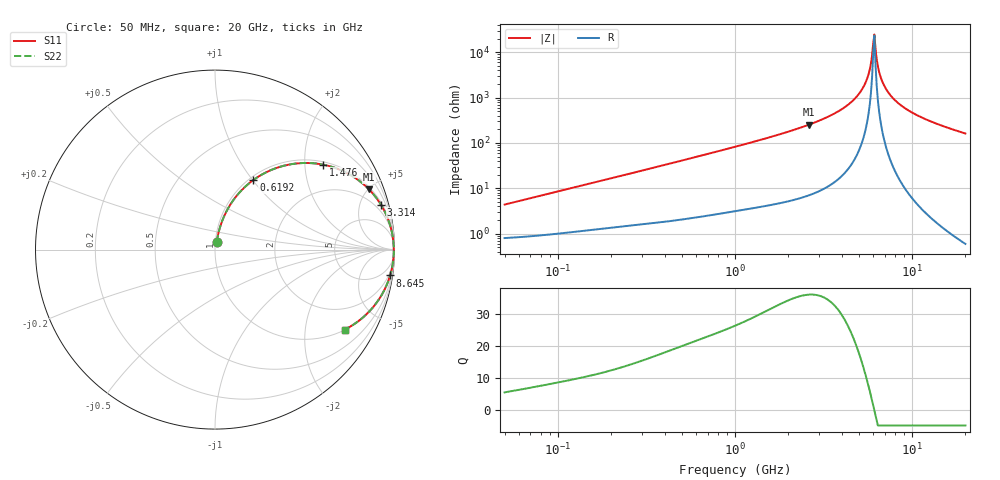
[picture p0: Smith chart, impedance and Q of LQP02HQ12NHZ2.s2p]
!Murata Part Number: LQP02HQ12NHZ2
!These Parameters are Measured in Series Mode Connection
!  o--[Z]--o
!Port1  Port2
!  o-------o
!Freq. Start=50[MHz] Stop=20[GHz], 401[Steps]
# Hz S RI R 50
!Freq.(Hz) S11(Real) S11(Imag) S21(Real) S21(Imag) S12(Real) S12(Imag) S22(Real) S22(Imag)
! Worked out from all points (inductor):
!   401 points, 50 MHz to 20 GHz, reference 50 ohm
!   read as one part in series: L = 13.6 nH near 51.52 MHz
!   highest Q = 36 at 2.608 GHz (marker M1), where L = 15.3 nH
!   self-resonance near 6.034 GHz
!   S11 on the Smith chart (normalised r, x): 50 MHz: 1.02, +0.09; 619.2 MHz: 1.05, +1.01; 1.476 GHz: 1.08, +2.49; 3.314 GHz: 1.21, +7.39; 8.645 GHz: 1, -14; 20 GHz: 1.01, -3.23
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5e7  0.00974 0.0423  0.9903 -0.0423  0.9903 -0.0423  0.00974 0.0423
1.364002e8  0.0238 0.1105  0.9762 -0.1105  0.9762 -0.1105  0.0238 0.1105
3.721004e8  0.0979 0.2696  0.9021 -0.2696  0.9021 -0.2696  0.0979 0.2696
6.192061e8  0.2136 0.3875  0.7864 -0.3875  0.7864 -0.3875  0.2136 0.3875
1e9  0.406 0.4724  0.594 -0.4724  0.594 -0.4724  0.406 0.4724
1.476162e9  0.604 0.473  0.396 -0.473  0.396 -0.473  0.604 0.473
2.608132e9  0.8566 0.3369  0.1434 -0.3369  0.1434 -0.3369  0.8566 0.3369
2.728004e9  0.8714 0.3211  0.1286 -0.3211  0.1286 -0.3211  0.8714 0.3211
3.314454e9  0.9256 0.2483  0.0744 -0.2483  0.0744 -0.2483  0.9256 0.2483
4.275624e9  0.9723 0.1466  0.0277 -0.1466  0.0277 -0.1466  0.9723 0.1466
5.117541e9  0.9901 0.0729  0.00994 -0.0729  0.00994 -0.0729  0.9901 0.0729
5.598765e9  0.9945 0.0358  0.00546 -0.0358  0.00546 -0.0358  0.9945 0.0358
5.769027e9  0.9954 0.0235  0.00461 -0.0235  0.00461 -0.0235  0.9954 0.0235
5.944466e9  0.9959 0.0111  0.00407 -0.0111  0.00407 -0.0111  0.9959 0.0111
6.125241e9  0.9962 -0.00131  0.00384 0.00131  0.00384 0.00131  0.9962 -0.00131
6.217679e9  0.9962 -0.00751  0.00385 0.00751  0.00385 0.00751  0.9962 -0.00751
6.503449e9  0.9957 -0.0261  0.00433 0.0261  0.00433 0.0261  0.9957 -0.0261
6.701223e9  0.9949 -0.0385  0.00505 0.0385  0.00505 0.0385  0.9949 -0.0385
7.442007e9  0.9899 -0.082  0.0101 0.082  0.0101 0.082  0.9899 -0.082
8.644534e9  0.9758 -0.144  0.0242 0.144  0.0242 0.144  0.9758 -0.144
1.220001e10  0.9091 -0.2834  0.0909 0.2834  0.0909 0.2834  0.9091 -0.2834
2e10  0.7217 -0.4463  0.2783 0.4463  0.2783 0.4463  0.7217 -0.4463
